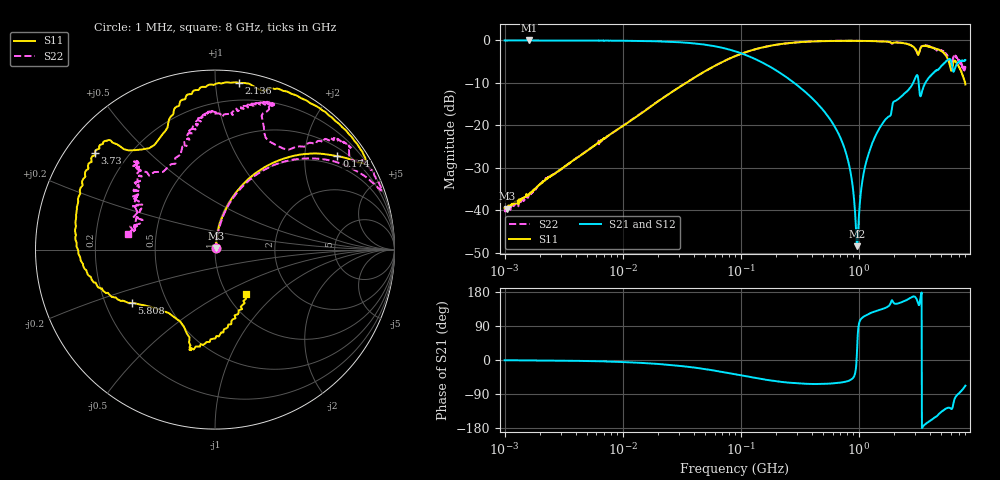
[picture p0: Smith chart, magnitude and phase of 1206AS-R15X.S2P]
!s-Parameter Generated by FASTRON Sdn. Bhd.
!FASTRON P/N : 1206AS-R15X
!Keysight Technologies: E5071C_MY46733604_B.14.02
!Date: Wed Nov 15 11:11:02 2023
!Version  :Rev00  Wed Nov 15 11:11:02 2023
!Data & Calibration Information:
!Freq  S11:SOLT2(ON)  S21:SOLT2(ON)  S12:SOLT2(ON)  S22:SOLT2(ON)
!PortZ  Port1:50+j0  Port2:50+j0
!When reading reference impedance value at option line is always used.
! Remarks : This data is being provided solely for informational purposes.
# Hz S dB R 50
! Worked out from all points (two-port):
!   1601 points, 1 MHz to 8 GHz, reference 50 ohm
!   highest |S21| = -0.04 dB at 1.614 MHz (marker M1); lowest = -48.4 dB at 968.6 MHz (marker M2)
!   |S21| within 3 dB of the highest: start of sweep to 100.4 MHz
!   lowest |S11| = -39.6 dB at 1.053 MHz (marker M3), VSWR 1.02, Z = 50.6 + j0.867 ohm
!   |S11| at or under -10 dB: start of sweep to 34.43 MHz; 7.965133 GHz to end of sweep
!   |S22| runs from -40.3 to -0.1 dB; largest |S21 - S12| = 0.0075
!   S11 on the Smith chart (normalised r, x): 1 MHz: 1.01, +0.02; 174 MHz: 0.71, +2.79; 2.136 GHz: 0.07, +1.15; 3.73 GHz: 0.09, +0.35; 5.808 GHz: 0.31, -0.27; 8 GHz: 1.21, -0.67
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1000000  -39.36 51.9  -0.04 -0.7  -0.06 -0.6  -39.55 57.0
1052806  -39.61 55.1  -0.04 -0.7  -0.06 -0.6  -39.71 56.1
1613744  -36.08 69.3  -0.04 -1.0  -0.05 -0.9  -36.29 66.4
4479405  -26.88 79.7  -0.07 -2.5  -0.07 -2.5  -26.88 80.5
2.00676e7  -14.29 76.9  -0.25 -10.5  -0.26 -10.4  -14.26 76.4
8.994653e7  -3.71 51.9  -2.59 -37.8  -2.59 -37.8  -3.72 49.9
1.740186e8  -1.34 37.5  -6.10 -53.4  -6.10 -53.4  -1.33 33.6
4.006501e8  -0.27 30.2  -13.56 -63.3  -13.57 -63.3  -0.27 21.0
7.480567e8  -0.12 36.9  -24.98 -58.2  -24.99 -58.2  -0.11 20.2
8.618919e8  -0.13 40.1  -31.86 -51.7  -31.86 -51.7  -0.11 21.0
9.68578e8  -0.13 43.3  -48.40 32.3  -48.50 32.6  -0.11 22.0
1.171668e9  -0.17 49.9  -28.01 118.8  -28.02 118.8  -0.17 24.3
1.7949e9  -0.40 69.6  -17.92 142.5  -17.94 142.3  -0.39 31.3
2.135779e9  -0.55 81.7  -13.93 149.1  -13.96 148.9  -0.51 37.3
2.750998e9  -1.14 99.3  -11.03 164.4  -11.06 164.2  -1.14 44.1
3.162936e9  -3.25 117.3  -8.54 151.0  -8.56 150.9  -3.35 55.9
3.406162e9  -1.47 133.8  -12.42 178.1  -12.45 177.9  -1.34 70.0
3.730463e9  -1.33 141.2  -9.60 -167.3  -9.61 -167.5  -1.26 70.6
4.856488e9  -2.32 179.7  -6.46 -140.1  -6.43 -140.3  -2.36 91.8
5.808211e9  -5.17 -147.4  -4.40 -126.0  -4.38 -126.4  -4.44 105.2
6.612025e9  -4.90 -102.1  -6.18 -97.6  -6.16 -98.1  -3.92 131.2
8e9  -10.38 -55.4  -4.65 -67.7  -4.64 -68.4  -6.16 169.9
